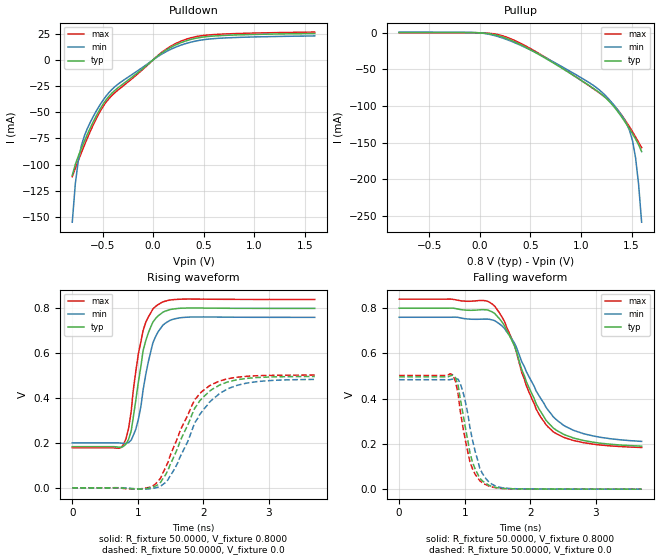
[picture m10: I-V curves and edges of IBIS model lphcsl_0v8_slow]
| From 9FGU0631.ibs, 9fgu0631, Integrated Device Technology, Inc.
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[Model]  lphcsl_0v8_slow
Model_type Output
Polarity   Non-Inverting
Enable   Active-High
Vmeas =  0.4000V
Cref =   2.0000pF
Rref =   0.0
Vref =   0.4000V
C_comp   1.1000pF   1.0000pF   1.2000pF
[Temperature Range]   25.0000   75.0000   0.0
[Voltage Range]   0.8000V   0.7600V   0.8400V
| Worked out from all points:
|   slope of the pulldown table from 0 to 0.12 V, typ, clamps not added: 13.7 ohm
|   slope of the pullup table from 0 to 0.12 V, typ, clamps not added: 63 ohm
|   rising waveform, R_fixture 50.0000, V_fixture 0.8000: 20-80 % time 218ps typ, 219ps min, 204ps max; typ from 0.183 V to 0.8 V
|   rising waveform, R_fixture 50.0000, V_fixture 0.0: 20-80 % time 486ps typ, 529ps min, 456ps max; typ from 0 V to 0.496 V
|   falling waveform, R_fixture 50.0000, V_fixture 0.8000: 20-80 % time 541ps typ, 598ps min, 517ps max; typ from 0.8 V to 0.19 V
|   falling waveform, R_fixture 50.0000, V_fixture 0.0: 20-80 % time 212ps typ, 216ps min, 198ps max; typ from 0.496 V to 0 V
[Pulldown]
|Voltage   I(typ)   I(min)   I(max)
-800mV    -110.2mA   -155mA     -111.5mA
-770mV    -99.93mA   -118.5mA   -103.7mA
-740mV    -91.85mA   -95.72mA   -96.19mA
-710mV    -84.57mA   -81.85mA   -88.81mA
-680mV    -77.65mA   -72.57mA   -81.59mA
-590mV    -58.63mA   -53.65mA   -61.5mA
-500mV    -43.03mA   -39.19mA   -45.27mA
-350mV    -26.89mA   -23.4mA    -29.01mA
100mV     7.489mA    6.294mA    8.221mA
340mV     18.58mA    16.02mA    20.1mA
670mV     23.16mA    20.72mA    24.52mA
1.6V      25.23mA    22.86mA    26.52mA
[Pullup]
|Voltage   I(typ)   I(min)   I(max)
-800mV    337.7uA    1.065mA    85.49uA
-50mV     204.4uA    529.3uA    54.19uA
220mV     -5.557mA   -6.902mA   -3.893mA
580mV     -29.32mA   -28.93mA   -27.89mA
1.15V     -78.54mA   -74.62mA   -79.03mA
1.27V     -92.39mA   -89.84mA   -91.65mA
1.36V     -107mA     -104.8mA   -104.8mA
1.48V     -131.4mA   -133.4mA   -128.6mA
1.51V     -138.1mA   -147.7mA   -135.4mA
1.54V     -145.2mA   -170.8mA   -142.4mA
1.57V     -153mA     -207.1mA   -149.6mA
1.6V      -162.5mA   -259mA     -157mA
[Ramp]
| variable   typ   min   max
dV/dt_r  0.2978/0.5152n   0.2899/0.5630n   0.3015/0.4866n
dV/dt_f  0.3658/0.5698n   0.3292/0.6363n   0.3934/0.5426n
R_load = 50.0000
[Rising Waveform]
R_fixture= 50.0000
V_fixture= 0.8000
V_fixture_min= 0.7600
V_fixture_max= 0.8400
|time   V(typ)   V(min)   V(max)
0s        183.3mV    200.3mV    178.8mV
780ps     184.6mV    198mV      192.6mV
860ps     216.2mV    202.3mV    265.5mV
900ps     254.7mV    212.6mV    342.8mV
1.01ns    474.3mV    307.4mV    600mV
1.08ns    610.9mV    434.7mV    700.5mV
1.23ns    738.5mV    646.3mV    797.5mV
1.31ns    767mV      695.9mV    816.9mV
1.68ns    801mV      759.2mV    841.3mV
3.7ns     800mV      760mV      839.9mV
[Rising Waveform]
R_fixture= 50.0000
V_fixture= 0.0
V_fixture_min= 0.0
V_fixture_max= 0.0
|time   V(typ)   V(min)   V(max)
0s        0V         0V         0V
970ps     -5.459mV   -4.255mV   -6.181mV
1.23ns    3.2mV      -2.436mV   8.688mV
1.35ns    25.22mV    7.227mV    44.19mV
1.46ns    77.52mV    35.76mV    113.1mV
1.61ns    178mV      111.6mV    224mV
1.87ns    355.6mV    290.1mV    393.4mV
2.17ns    445.4mV    401.8mV    466.2mV
2.65ns    487.4mV    466.1mV    496.9mV
3.7ns     496.3mV    483.2mV    502.5mV
[Falling Waveform]
R_fixture= 50.0000
V_fixture= 0.8000
V_fixture_min= 0.7600
V_fixture_max= 0.8400
|time   V(typ)   V(min)   V(max)
0s        800mV      760mV      840mV
1.38ns    788.8mV    750.7mV    826.2mV
1.57ns    739mV      721.6mV    760.7mV
1.72ns    657.6mV    664mV      663.5mV
1.94ns    475.7mV    520.1mV    458mV
2.13ns    357mV      415.2mV    333mV
2.28ns    291.9mV    346.8mV    273.1mV
2.5ns     243.8mV    284mV      230.5mV
2.8ns     216mV      246.5mV    206.3mV
3.7ns     190.3mV    211.3mV    184.4mV
[Falling Waveform]
R_fixture= 50.0000
V_fixture= 0.0
V_fixture_min= 0.0
V_fixture_max= 0.0
|time   V(typ)   V(min)   V(max)
0s        496.5mV    483.9mV    502.6mV
820ps     504mV      486.8mV    505.5mV
900ps     457.7mV    486.2mV    420mV
930ps     403.3mV    468.9mV    350.5mV
1.01ns    273.4mV    387.5mV    216.5mV
1.08ns    161.4mV    272.8mV    120.6mV
1.23ns    48.64mV    92.76mV    37.35mV
1.31ns    27.86mV    51.96mV    21.44mV
1.68ns    2.03mV     3.194mV    1.694mV
3.7ns     74.09uV    113uV      58.19uV
